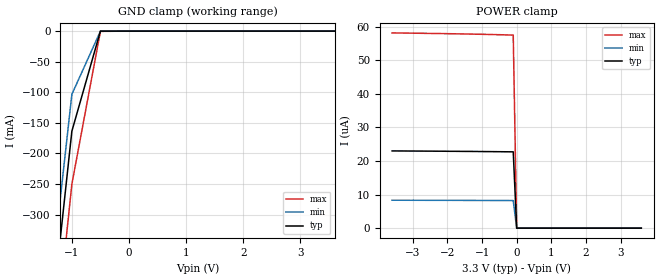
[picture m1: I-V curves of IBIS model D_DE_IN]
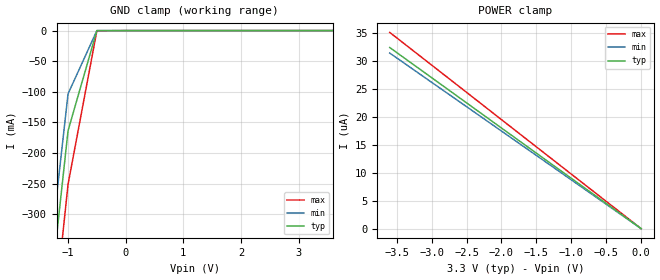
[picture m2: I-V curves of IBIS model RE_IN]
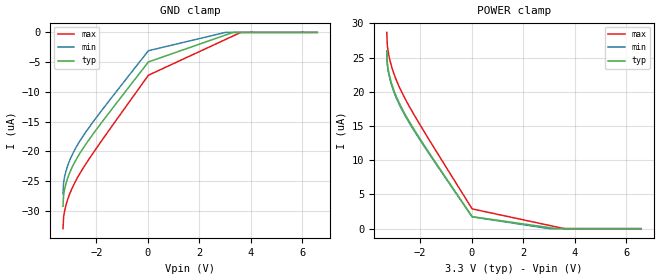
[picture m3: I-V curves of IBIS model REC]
| Texas Instruments Incorporated
| 3.3v Full-Duplex RS-485 Drivers and Receivers
| Model valid for speed grades upto 26Mbps(13MHz Clock frequency)
| Marketing part#   Voltage Range   Package-type   Temperature
| SN65HVD34DR   3.0V - 3.6V   SOIC (D) 14-pin  -40C to 85C
[IBIS Ver]   4.0
[Comment char]   |_char
[File name]   sn65hvd34.ibs
[File Rev]   1.0
[Date]   05/04/2010
[Source]   Model built from TISPICE simulations at:
   Texas Instruments Incorporated.
   Analog-eLab, HPA
   12500 TI Blvd
   Dallas, TX -75243
   For Support e-mail: elab_scm_ibis@list.ti.com
[Notes]
   Rev 1.0: 12/06/2010
   - New simulations for DRVR, and REC model characteristics
   - DRVR pullup and pulldown non-montonicity reflects true buffer behavior.
   - HVD33 requires that the device never exceed more than 250 mA of
   current during a short-circuit event with a specific rise time.
   - C_comp although listed in numberical order of value are obtained from varying PVT conditions.
   For PVT conditions for eachspecific value, refer to the buffer description under repective [Model].
   IBIS model user is responsible for using appropriate C_comp to simulate for Signal Integrity.
[Disclaimer] This product is designed as an aid for customers of Texas Instruments.
   No warranties, either expressed or implied, with respect to this third
   party software (if any) or with respect to its fitness for any
   particular purpose is claimed by Texas Instruments or the author. The
   software (if any) is provided solely on an "as is" basis. The entire
   risk as to its quality and performance is with the customer
[Copyright]   (C)Copyright 2010 Texas Instruments Incorporated.
   All rights reserved.
[Component]   HVD33D
[Manufacturer]  Texas Instruments Incorporated
[Package]
|   typ   min   max
R_pkg   0.071   0.050   0.091
L_pkg   2.203nH   1.540nH   2.930nH
C_pkg   0.465pF   0.385pF   0.609pF
[Pin]   signal_name   model_name   R_pin   L_pin   C_pin
2   R   RECEIVER_OUT   0.076   2.346n   0.483p
3   RE   RE_IN   0.072   1.934n   0.404p
4   DE   D_DE_IN   0.053   1.585n   0.397p
5   D   D_DE_IN   0.062   1.755n   0.395p
6   GND   GND   0.090   2.593n   0.498p
7   GND   GND   0.072   2.930n   0.608p
9   Y   DRVR   0.073   2.300n   0.480p
10   Z   DRVR   0.076   2.012n   0.407p
11   A   REC   0.070   1.897n   0.412p
12   B   REC   0.050   1.540n   0.385p
13   VCC   POWER   0.091   2.615n   0.500p
14   VCC   POWER   0.073   2.929n   0.609p
[Diff_pin]   inv_pin   vdiff   tdelay_typ   tdelay_min   tdelay_max
| The 'A' pin is Diff_pin and the 'B' pin is the inv_pin
9   10   0.200   0 0 0
11   12   0.200   0 0 0
| Models and submodels in the file (5): D_DE_IN (Input), RE_IN (Input), REC (Input), DRVR (3-state), RECEIVER_OUT (Output)
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|   Driver Input / Driver Enable / Model
[Model]   D_DE_IN
Model_type   Input
|Signals   D,DE
Vinh = 2.0
Vinl = 0.8
|   typ   min   max
|   (nom PVT)   (slow PVT)   (fast PVT)
C_comp   7.8pF   7.3pF   8.1pF
|   typ   min   max
[Temperature Range]   27   -40   85
[Voltage range]   3.3V   3.0V   3.6V
[GND_clamp]
|   Voltage   I(typ)   I(min)   I(max)
-3.6V     -2.348A    -2.232A    -2.506A
-1.5V     -596.3mA   -523.6mA   -696.4mA
-1V       -163.5mA   -103.3mA   -250mA
-500mV    -12.8uA    -27.56uA   -399.4uA
3.6V      22.76uA    57.48uA    8.245uA
[Power_clamp]
| Note that the[POWER_clamp]voltage table is referenced to Vcc
| and is calculated using Vtable=Vcc - Vmeasured.
|   Voltage   I(typ)   I(min)   I(max)
-3.6V     23.01uA    8.325uA    58.18uA
-100mV    22.74uA    8.227uA    57.52uA
0V        0A         0A         0A
3.6V      0A         0A         0A
|   Receiver Enable / Model
[Model]   RE_IN
Model_type   Input
|Signals   RE
Vinh = 2.0
Vinl = 0.8
|   typ   min   max
|   (nom PVT)   (slow PVT)   (fast PVT)
C_comp   7.8pF   7.3pF   8.1pF
|   typ   min   max
[Temperature Range]   27   -40   85
[Voltage range]   3.3V   3.0V   3.6V
[GND_clamp]
|   Voltage   I(typ)   I(min)   I(max)
-3.6V     -2.348A    -2.232A    -2.508A
-1.5V     -596.4mA   -523.7mA   -697.7mA
-1V       -163.6mA   -103.4mA   -251.3mA
-500mV    -35.38uA   -43.24uA   -430.8uA
3.6V      2.698uA    15.58pA    5.231uA
[Power_clamp]
| Note that the[POWER_clamp]voltage table is referenced to Vcc
| and is calculated using Vtable=Vcc - Vmeasured.
|   Voltage   I(typ)   I(min)   I(max)
-3.6V     32.37uA    31.38uA    35.07uA
-3.3V     29.67uA    28.77uA    32.15uA
-3V       26.98uA    26.15uA    29.23uA
-2.5V     22.48uA    21.8uA     24.36uA
-2V       17.98uA    17.44uA    19.48uA
-1.5V     13.49uA    13.08uA    14.61uA
-1V       8.992uA    8.718uA    9.742uA
-500mV    4.496uA    4.359uA    4.871uA
0V        0A         0A         0A
|   Receiver Input / Model
[Model]   REC
Model_type   Input
|Signals   A,B
Vinh = 2.0
Vinl = 0.8
|   typ   min   max
C_comp   116.75fF   116.7fF   116.8fF
|   typ   min   max
[Temperature Range]   27   -40   85
[Voltage range]   3.3V   3.0V   3.6V
[GND_clamp]
|   Voltage   I(typ)   I(min)   I(max)
-3.3V     -29.21uA   -27.1uA    -32.99uA
-3.275V   -27.31uA   -25.21uA   -31.03uA
-3.226V   -26.14uA   -24.04uA   -29.79uA
-3.176V   -25.3uA    -23.21uA   -28.92uA
-3.003V   -23.22uA   -21.14uA   -26.76uA
-2.731V   -20.94uA   -18.87uA   -24.37uA
-1.964V   -16.1uA    -14.08uA   -19.23uA
16.5mV    -4.966uA   -3.081uA   -7.2uA
3.011V    -448nA     0A         -1.192uA
3.308V    0A         0A         -595.9nA
3.605V    0A         0A         0A
6.575V    0A         0A         0A
[POWER Clamp]
|   Voltage   I(typ)   I(min)   I(max)
-3.3V     26uA       25.74uA    28.67uA
-3.275V   24.1uA     23.85uA    26.71uA
-3.226V   22.92uA    22.68uA    25.48uA
-3.176V   22.08uA    21.85uA    24.61uA
-3.003V   20.01uA    19.79uA    22.44uA
-2.731V   17.72uA    17.51uA    20.05uA
-2.409V   15.55uA    15.36uA    17.76uA
-1.939V   12.72uA    12.56uA    14.74uA
16.5mV    1.754uA    1.725uA    2.888uA
3.011V    158.2nA    0A         478.1nA
3.605V    0A         0A         0A
6.575V    0A         0A         0A
